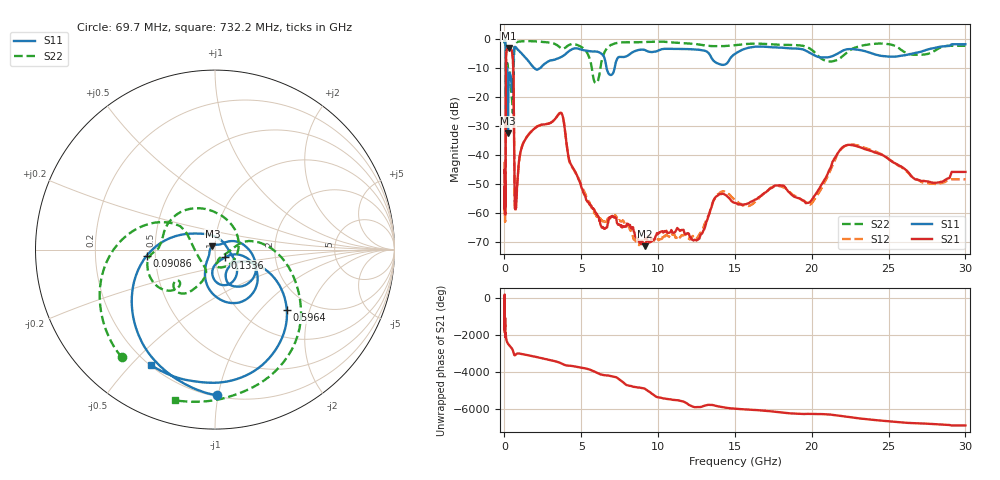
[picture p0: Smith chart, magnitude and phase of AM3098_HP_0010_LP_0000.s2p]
! Date/Time: Thu, Feb 28, 2019 8:32 AM
! Network Analyzer: Agilent Technologies E8364B Rev: A.07.50.67
! Sweep from 0.010 to 30.000 GHz, 1601 Points, Sweep Type: LOG
! Power Supply: 5.022 V, 0.002 A
# Hz S DB R 50
!freq MagS11 AngS11 MagS21 AngS21 MagS12 AngS12 MagS22 AngS22
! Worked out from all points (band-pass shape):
!   1601 points, 10 MHz to 30 GHz, reference 50 ohm
!   highest |S21| = -2.95 dB at 266.5 MHz (marker M1); lowest = -71.5 dB at 9.118 GHz (marker M2)
!   |S21| within 3 dB of the highest: 106.3 MHz to 533.8 MHz (427.6 MHz wide, 134 % of centre)
!   lowest |S11| = -32.5 dB at 228.2 MHz (marker M3), VSWR 1.05, Z = 48.5 + j1.8 ohm
!   |S11| at or under -10 dB: 175.9 MHz to 562.1 MHz (386.2 MHz wide, 105 % of centre); 1.957 GHz to 2.281 GHz (323.8 MHz wide, 15.3 % of centre); 6.65 GHz to 7.166 GHz (516.3 MHz wide, 7.47 % of centre)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
!   |S22| runs from -25.5 to -0.5 dB; largest |S21 - S12| = 0.01
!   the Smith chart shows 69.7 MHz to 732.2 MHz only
!   S11 on the Smith chart (normalised r, x): 69.7 MHz: 0.21, -0.99; 90.86 MHz: 0.45, -0.04; 133.6 MHz: 1.11, -0.10; 596.4 MHz: 1.53, -1.43; 732.2 MHz: 0.20, -0.57
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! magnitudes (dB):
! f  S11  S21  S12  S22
! 10 MHz  -0.4  -46.2  -42.2  -0.5
! 38.04 MHz  -0.5  -59.6  -62.5  -0.8
! 69.7 MHz  -1.8  -54.9  -52.4  -2.0
! 90.86 MHz  -8.4  -18.6  -18.7  -10.3
! 99.92 MHz  -24.1  -7.9  -7.9  -17.7
! 133.6 MHz  -23.1  -3.8  -3.7  -11.5
! 144.7 MHz  -14.0  -3.5  -3.5  -10.3
! 187.7 MHz  -11.6  -3.4  -3.4  -8.3
! 228.2 MHz  -32.5  -3.0  -3.0  -10.0
! 266.5 MHz  -15.2  -2.9  -2.9  -10.5
! 550.5 MHz  -11.9  -7.2  -7.2  -25.3
! 596.4 MHz  -5.6  -17.1  -17.0  -10.9
! 665.8 MHz  -2.6  -55.5  -55.9  -2.3
! 732.2 MHz  -2.7  -58.5  -57.1  -1.2
! 2.084 GHz  -10.5  -30.3  -30.2  -0.7
! 3.686 GHz  -6.1  -25.5  -25.4  -3.0
! 5.959 GHz  -4.2  -60.0  -60.9  -15.1
! 7.926 GHz  -5.9  -64.8  -64.3  -1.0
! 9.118 GHz  -3.6  -71.5  -69.2  -1.0
! 19.8 GHz  -4.4  -56.5  -56.8  -3.0
! 22.67 GHz  -3.4  -36.6  -36.4  -3.2
! 30 GHz  -1.7  -45.9  -48.4  -2.2
